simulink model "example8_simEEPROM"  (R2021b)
settings: Solver=FixedStepAuto  StartTime=0  StopTime=inf  FixedStep=0.5  RelTol=1e-3  EnableMultiTasking=on
undefined symbols (not defined in the file or in its folder): based, classic, dsPic33, MCC, Microchip, PIC24
libraries: embeddedCreatorLib x6, simEEPROMLib x4, emMBSlaveLib x1

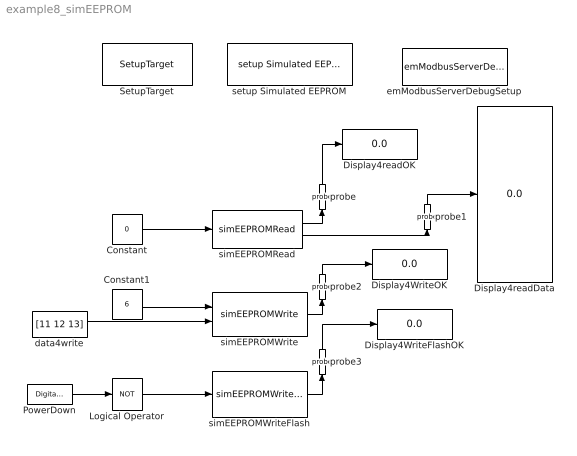
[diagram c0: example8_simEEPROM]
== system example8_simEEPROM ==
  Constant : Constant  Value=0  OutDataTypeStr=uint16
  Constant1 : Constant  Value=6  OutDataTypeStr=uint16
  Display4WriteFlashOK : Display
  Display4WriteOK : Display
  Display4readData : Display
  Display4readOK : Display
  Logical Operator : Logic  Operator=NOT  AllPortsSameDT=off  OutDataTypeStr=boolean
  PowerDown : embeddedCreatorLib/Digital Input  c_Name_method=By physical port name and bit number  c_PortName=B  c_BitNo=6  c_DinAccessName="\"PORTBbits.RB6\""  c_EnableFilter=on  c_Filter_method=Continuous sample multiple times in one sample period  c_filterQTY=8  c_initialV=1  c_sampleTime=-1
  SetupTarget : embeddedCreatorLib/SetupTarget  Tag=SetupTarget  Priority=0  c_platform=Microchip PIC24/dsPic33 based on MCC classic  c_debug=on
  data4write : Constant  Value=[11 12 13]  OutDataTypeStr=uint8
  emModbusServerDebugSetup : emMBSlaveLib/emModbusServerDebugSetup  Tag=emModbusSlaveSetup  c_objID=0  c_uartNo=2  c_baudrate=19200  c_serverID=1  c_baudrate4PC=19200  c_forceLongerSpace=on  c_holdingRegsQTY=1000  c_minHoldingAddr=789  c_inputRegsQTY=200  c_minInputRegAddr=20  c_coilRegsQTY=300  c_minCoilAddr=30  c_discreteRegsQTY=400  c_minDiscreteAddr=40  c_enableDebug=on  c_breakpointMaxQTY=100  c_probeMaxWordQTY=200  c_emWaitQTY=0  g_COMPortNo=COM5  c_Name_method=By physical port name and bit number  c_PortName=B  c_BitNo=11  c_TxEnable485="\"LATBbits.LATB11\""  c_TxEnable485Polarity=on
  probe : embeddedCreatorLib/probe  Tag=emProbe  c_ObjID=1  c_serverID=1  c_UartNo=1  c_StartAddr=11  c_ConstantDataSource=off
  probe1 : embeddedCreatorLib/probe  Tag=emProbe  c_ObjID=0  c_serverID=1  c_UartNo=1  c_StartAddr=2  c_ConstantDataSource=off
  probe2 : embeddedCreatorLib/probe  Tag=emProbe  c_ObjID=2  c_serverID=1  c_UartNo=1  c_StartAddr=12  c_ConstantDataSource=off
  probe3 : embeddedCreatorLib/probe  Tag=emProbe  c_ObjID=3  c_serverID=1  c_UartNo=1  c_StartAddr=13  c_ConstantDataSource=off
  setup Simulated EEPROM : simEEPROMLib/setup Simulated EEPROM  Tag=SimulatedEEPROM  Priority=0  c_doublewrite=on  c_EEPROMSize=256  c_initialData=[0 0 1 24]  c_initalDataType=[uint8 uint8 uint8 uint8]
  simEEPROMRead : simEEPROMLib/simEEPROMRead  c_DataType=uint8  c_DataDimension=9  c_sampleTime=-1
  simEEPROMWrite : simEEPROMLib/simEEPROMWrite  c_sampleTime=-1
  simEEPROMWriteFlash : simEEPROMLib/simEEPROMWriteFlash  c_sampleTime=-1
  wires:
  Constant/1 -> simEEPROMRead/1
  PowerDown/1 -> Logical Operator/1
  Logical Operator/1 -> simEEPROMWriteFlash/1
  Constant1/1 -> simEEPROMWrite/1
  data4write/1 -> simEEPROMWrite/2
  probe/1 -> Display4readOK/1
  simEEPROMRead/1 -> probe/1
  simEEPROMRead/2 -> probe1/1
  probe1/1 -> Display4readData/1
  simEEPROMWrite/1 -> probe2/1
  simEEPROMWriteFlash/1 -> probe3/1
  probe2/1 -> Display4WriteOK/1
  probe3/1 -> Display4WriteFlashOK/1
